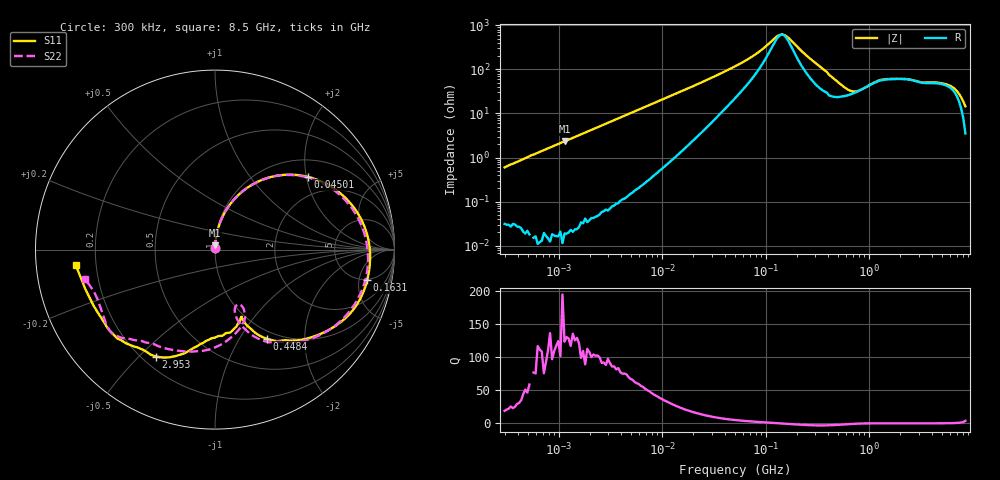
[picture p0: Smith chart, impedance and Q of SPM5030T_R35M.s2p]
! S-Parameter Data Generated by TDK Corporation
! Copyright(C) 2023 TDK Corporation.
! All Rights Reserved.
! TDK P/N: SPM5030T-R35M (Inductor)
! Property: L=350nH at 100kHz
! Size(LxWxT): 5.2x5x3mm
! Model Type: s2p (Touchstone File Format Version 1.0)
! Frequency: DC=Yes Start=0.3MHz Stop=8500MHz 225points Log-sweep
! Model Generated on Sep. 29, 2023
! Port Assignments:
!  1 ---@@@--- 2
! Applicable Conditions:
!  Temperature = 25 degC
!  DC Bias Current = 0 A
!  Small Signal Operation
! Terms and conditions regarding TDK Simulation Models
! (1)This simulation model is being provided solely for informational purposes. Please refer to the specifications of the products in terms of detailed characteristics of such products.
! (2)In no event shall TDK Corporation of any of its subsidiaries be liable for any loss or damage arising, directly or indirectly,
!  From any information contained in this simulation model, including, but not limited to loss or damages arising from any inaccuracies, omissions or errors in connection with such information.
! (3)Any and all copyrights on this simulation model are owned by TDK Corporation.
!  Duplication or redistribution of this simulation model without prior written permission from TDK Corporation is prohibited.
! (4)This simulation model is subject to any modification or change without any prior notice.
! (5)Neither TDK Corporation nor any of its subsidiaries shall make any warranty, express or implied,
!  Including but not limited to the correctness, implied warranties of merchantability and fitness for a particular purpose with respect to this simulation models.
! (6)The use of this simulation model shall be deemed to have consented to the terms and conditions hereof.
# Hz S MA R 50
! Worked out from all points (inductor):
!   224 points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, 300 kHz to 8.5 GHz, reference 50 ohm
!   read as one part in series: L = 322 nH near 314.1 kHz
!   highest Q = 128 at 1.138 MHz (marker M1), where L = 325 nH
!   self-resonance near 143.8 MHz
!   S11 on the Smith chart (normalised r, x): 300 kHz: 1.00, +0.01; 45.01 MHz: 1.43, +2.03; 163.1 MHz: 4.85, -6.54; 448.4 MHz: 0.89, -1.32; 2.953 GHz: 0.25, -0.56; 8.5 GHz: 0.12, -0.05
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300000  0.006582 91.0  0.9999 -0.4  0.9982 -0.2  0.006704 92.7
1137941  0.02309 88.3  0.9997 -1.4  0.9991 -1.3  0.02313 88.4
1721110  0.03466 87.4  0.9993 -2.1  0.9987 -2.0  0.03468 87.5
9430415  0.1853 77.2  0.9774 -11.2  0.9776 -11.1  0.1857 77.3
2.060362e7  0.3813 63.0  0.9004 -23.5  0.9005 -23.3  0.3822 63.0
4.501492e7  0.6561 38.2  0.6536 -42.5  0.6537 -42.3  0.6549 37.8
5.167171e7  0.6998 33.1  0.5897 -45.7  0.5898 -45.6  0.6974 32.7
8.182903e7  0.8131 15.9  0.3569 -52.4  0.3569 -52.2  0.8047 15.1
1.356836e8  0.8657 -3.7  0.1426 -18.1  0.1427 -17.9  0.8557 -5.0
1.630757e8  0.8649 -11.3  0.1584 17.8  0.1585 17.9  0.8529 -12.9
2.831228e8  0.7651 -36.8  0.4434 33.2  0.4435 33.3  0.7534 -39.3
3.562888e8  0.6798 -48.1  0.5655 24.0  0.5657 24.2  0.6638 -51.1
4.483627e8  0.575 -59.8  0.6725 11.1  0.6725 11.2  0.5531 -64.0
6.185683e8  0.4482 -67.6  0.7222 -7.4  0.7223 -7.2  0.4016 -72.4
8.533868e8  0.4024 -68.3  0.684 -25.7  0.684 -25.6  0.3307 -68.1
1.232735e9  0.4592 -77.4  0.5597 -42.5  0.56 -42.3  0.4101 -65.8
1.551304e9  0.4908 -90.2  0.4952 -50.3  0.4954 -50.1  0.4871 -77.4
2.044041e9  0.545 -100.2  0.4349 -61.1  0.435 -61.0  0.5672 -96.6
2.952659e9  0.6804 -118.8  0.3596 -77.8  0.3597 -77.6  0.6239 -120.3
5.884306e9  0.7409 -144.5  0.2171 -111.6  0.217 -111.4  0.7382 -143.8
7.072242e9  0.745 -155.1  0.2046 -123.7  0.2046 -123.5  0.7151 -152.9
8.5e9  0.781 -173.8  0.1671 -140.3  0.1678 -140.4  0.744 -167.2
